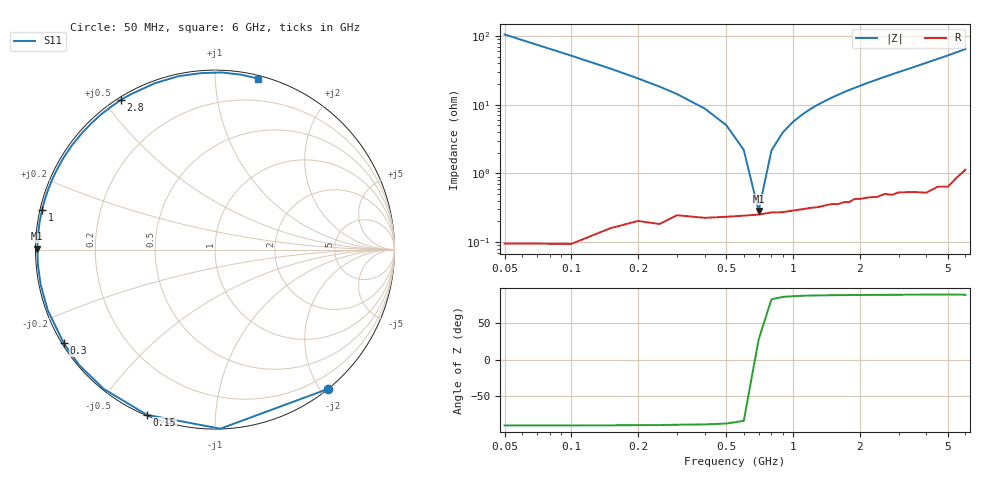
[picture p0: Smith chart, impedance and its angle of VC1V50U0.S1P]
! Infineon Technologies  Discrete & RF Semiconductors
! BBY 56-03
! Si Tuning Diode in SOD323
! VR = 1.5 V
! S-Parameters:  June  1999
# GHz  S  MA  R  50
!  f  S11
! GHz  MAG  ANG
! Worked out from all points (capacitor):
!   34 points, 50 MHz to 6 GHz, reference 50 ohm
!   read as one part to ground: C = 30.2 pF near 50 MHz
!   lowest |Z| = 284 mohm at 700 MHz (marker M1)
!   series resonance near 694.3 MHz, so ESL is about 1.7 nH
!   S11 on the Smith chart (normalised r, x): 50 MHz: 0.00, -2.10; 150 MHz: 0.00, -0.67; 300 MHz: 0.00, -0.28; 1 GHz: 0.01, +0.11; 2.8 GHz: 0.01, +0.55; 6 GHz: 0.02, +1.28
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0.05  0.9993 -51.0
0.1  0.9982 -88.3
0.15  0.9956 -112.4
0.2  0.9934 -128.6
0.25  0.9935 -139.8
0.3  0.9909 -148.2
0.4  0.9913 -160.1
0.5  0.9908 -168.5
0.6  0.9903 -175.0
0.7  0.99 179.7
0.8  0.9892 175.1
1  0.9887 167.2
1.1  0.9883 163.7
1.3  0.9876 157.3
1.5  0.9866 151.5
1.6  0.9868 148.9
1.8  0.9862 143.7
2  0.9852 139.0
2.2  0.9849 134.4
2.4  0.9851 130.2
2.8  0.9851 122.2
3  0.9845 118.5
3.5  0.9857 109.9
4  0.9875 101.8
4.5  0.9863 94.4
5  0.9878 87.8
5.5  0.9852 81.4
6  0.9831 75.8
